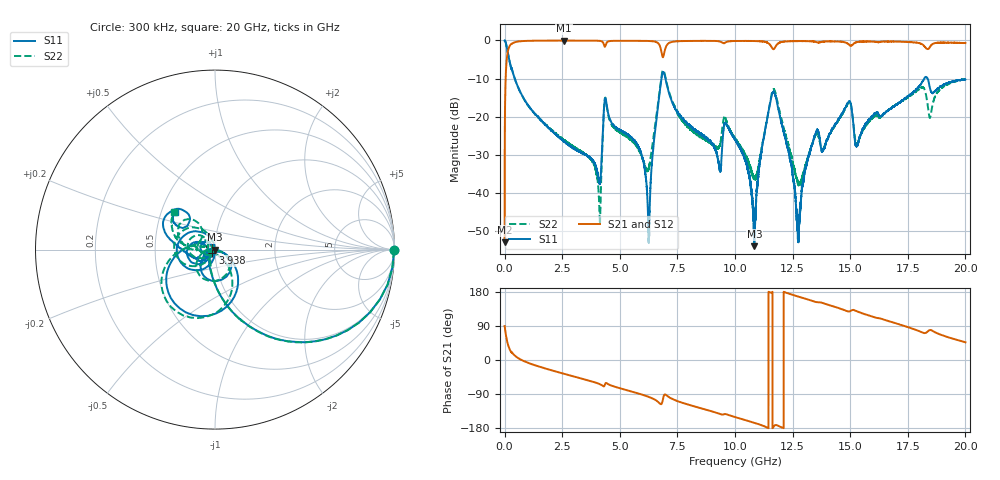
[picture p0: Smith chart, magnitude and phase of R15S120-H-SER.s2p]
!{R15S120}
!Johanson Technology Inc.
!www.johansontechnology.com
!Test Board Conditions:
!Substrate Type  RO4350B
!Substrate Thickness  20 mil
!Substrate Dk  3.66
!TL Type: GCPW
!TL Trace Width  34 mil
!TL Gap  10 mil
!Electrode orientation  Horizontal
!DUT TOPOLOGY	SERIES
!Mounting Pad LxW  26x52 mil
! Created Sat Feb  6 14:08:57 2021
# hz S ma R 50
! 2 Port Network Data from SP1.SP block
! freq  magS11  angS11  magS21  angS21  magS12  angS12  magS22  angS22
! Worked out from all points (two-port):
!   20001 points, 300 kHz to 20 GHz, reference 50 ohm
!   highest |S21| = -0.03 dB at 2.578 GHz (marker M1); lowest = -53.0 dB at 300 kHz (marker M2)
!   |S21| within 3 dB of the highest: 136.1 MHz to 6.809 GHz (6.673 GHz wide, 192 % of centre); 6.937 GHz to end of sweep
!   lowest |S11| = -54.1 dB at 10.84 GHz (marker M3), VSWR 1.00, Z = 49.8 - j0.0425 ohm
!   |S11| at or under -10 dB: 440.3 MHz to 6.807 GHz (6.367 GHz wide, 176 % of centre); 6.98 GHz to 18.22 GHz (11.24 GHz wide, 89.2 % of centre); 18.36 GHz to end of sweep
!   |S22| runs from -48.4 to 0.0 dB; largest |S21 - S12| = 0.014
!   S11 on the Smith chart (normalised r, x): 300 kHz: open; 3.938 GHz: 0.97, -0.03; 20 GHz: 0.59, +0.28
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300000  0.9979 -0.3  0.002241 89.6  0.002153 89.3  0.9972 -0.3
1.053e8  0.7878 -39.5  0.6113 50.3  0.6129 50.2  0.7884 -39.5
2.263e8  0.5139 -62.3  0.8529 27.3  0.8529 27.2  0.5146 -62.4
2.5783e9  0.0471 -129.0  0.9967 -36.4  0.9955 -36.4  0.04935 -122.5
3.3343e9  0.0337 -133.6  0.9947 -49.0  0.9951 -49.0  0.03464 -140.4
3.9383e9  0.02315 -129.1  0.9928 -59.4  0.9929 -59.5  0.021 -157.0
4.1323e9  0.01307 -79.1  0.988 -63.7  0.9872 -63.7  0.003982 -107.8
4.4073e9  0.1594 -112.9  0.9061 -60.5  0.9065 -60.4  0.1574 -128.4
5.8533e9  0.03747 -179.9  0.9896 -89.3  0.99 -89.3  0.03492 -165.5
6.2523e9  0.002415 91.7  0.9853 -97.3  0.9851 -97.2  0.02051 -94.1
6.6673e9  0.1425 -39.4  0.9189 -110.9  0.9173 -110.9  0.1556 -55.6
6.9043e9  0.381 -121.6  0.6344 -95.4  0.6338 -95.3  0.4019 -128.0
9.3153e9  0.02248 142.5  0.9724 -141.8  0.9744 -141.9  0.03988 179.1
9.5843e9  0.08277 164.6  0.94 -142.7  0.9422 -142.8  0.0955 153.4
1.00003e10  0.0503 129.9  0.9826 -150.6  0.9839 -150.6  0.05146 126.7
1.08403e10  0.001982 -167.6  0.9817 -165.7  0.9812 -165.7  0.01563 171.5
1.16473e10  0.21 -167.1  0.7724 -178.5  0.7732 -178.6  0.2233 -176.6
1.27373e10  0.003678 149.5  0.979 167.6  0.9802 167.5  0.01323 152.7
1.33343e10  0.04194 -114.8  0.9736 156.5  0.9749 156.4  0.04213 -140.6
1.49273e10  0.1553 -160.4  0.8956 128.2  0.8919 128.1  0.1514 176.7
1.66673e10  0.1213 -157.4  0.9718 102.6  0.9618 102.6  0.1225 -179.8
2e10  0.3073 136.2  0.9236 46.7  0.9164 46.5  0.3101 137.5
